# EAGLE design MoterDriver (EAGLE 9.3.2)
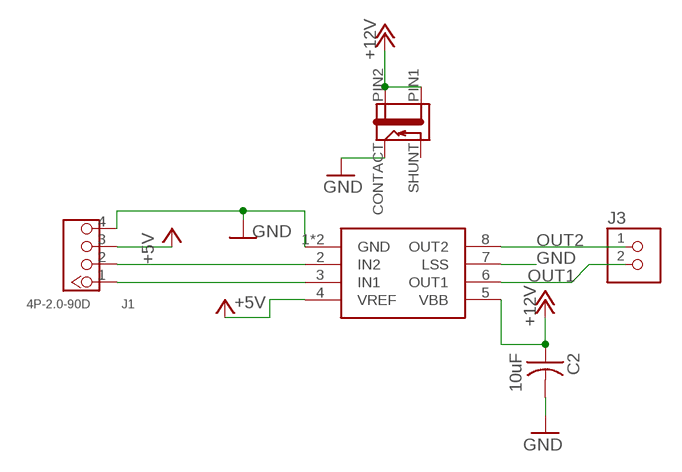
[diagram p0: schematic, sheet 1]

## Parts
C2  10uF  CAP-US1206FAB  [C1206FAB]
J1  4P-2.0-90D  GROVE-CONNECTOR-DIP-90D(4P-2.0)  [HW4-2.0-90D]
J2  JACK-2.1MM  [PJ-002AH-SMT]
J3  TERM-1X02-FABLAB  [ED555DS-2DS]
U$2  A4953-H-BRIDGE-MOTOR-DRIVER-PAD  [SOIC8_PAD]

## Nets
+5V: J1.3 U$2.4(VREF)
+12V: C2.1 J2.PIN1 J2.PIN2 U$2.5(VBB)
GND: C2.2 J1.4 J2.CONTACT U$2.1(GND) U$2.7(LSS) U$2.GND
OUT1: J3.2 U$2.6(OUT1)
OUT2: J3.1 U$2.8(OUT2)
PIN1: J1.1 U$2.3(IN1)
PIN2: J1.2 U$2.2(IN2)

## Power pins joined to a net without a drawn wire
SHUNT: J2.SHUNT

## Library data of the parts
C2 = fab:CAP-US
J1 = OPL_Connector:GROVE-CONNECTOR-DIP-90D(4P-2.0): 320110034
J2 = fab:JACK-2.1MM: SMD DC power jack PJ-002AH-SMT As found in the fablab inventory. Made by Zaerc.
J3 = fab:TERM-1X02: 3.5mm terminal block, 2 positions ED555-2DS as found in the fablab inventory.
U$2 = fab:A4953-H-BRIDGE-MOTOR-DRIVER-PAD

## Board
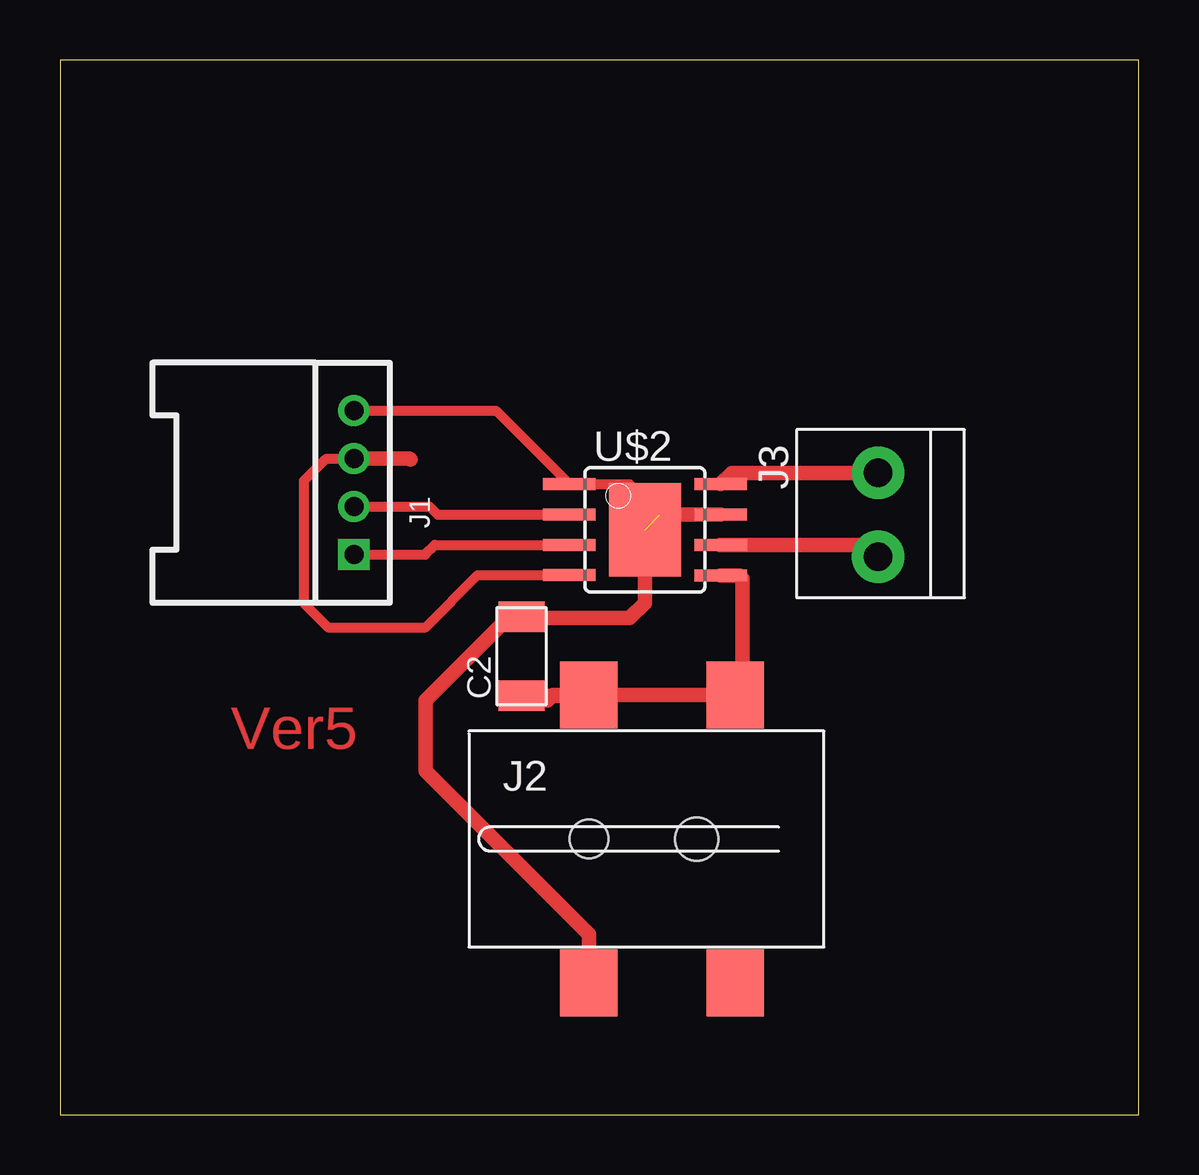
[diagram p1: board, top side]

Size 44.97 x 43.97 mm. Coordinates in mm from the lower left corner, seen from the top.
Outline: 0,0 44.97,0 44.97,43.97 0,43.97 0,0
Copper layers (1*16): Top 0.035mm / dielectric 1.5mm / Bottom 0.035mm
Design rules "default": minimum track width 6mil, minimum drill 0.35mm, track to track 6mil, track to pad 6mil, pad to pad 6mil, via to via 6mil, smd to smd 6mil, copper to edge 40mil, drill to drill 6mil, minimum pad ring 10mil, minimum via ring 8mil, stop-mask expansion 4mil, vias tented up to drill 0mil, thermal gap 10mil

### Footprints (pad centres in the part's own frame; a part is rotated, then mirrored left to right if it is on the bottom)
C1206FAB = smd 1.27 x 1.905: 1 -1.651,0; 2 1.651,0
HW4-2.0-90D = drill 0.8 pad 1.27 square: 1 -3,0 | drill 0.8 pad 1.27: 2 -1,0; 3 1,0; 4 3,0
PJ-002AH-SMT = smd 2.4 x 2.8: CONTACT -2.4,-6; PIN1 3.7,6; PIN2 -2.4,6; SHUNT 3.7,-6 | hole 1.6: -2.4,0 | hole 1.8: 2.1,0
ED555DS-2DS = drill 1.2 pad 2.184: 1 1.8,0; 2 -1.7,0
SOIC8_PAD = smd 0.5 x 2.2: 1 -1.905,-3.154; 2 -0.645,-3.154; 3 0.625,-3.154; 4 1.895,-3.154; 5 1.905,3.154; 6 0.635,3.154; 7 -0.635,3.154; 8 -1.905,3.154 | smd 3.886 x 2.997: GND 0,0

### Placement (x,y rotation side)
C2  19.24,19.11 90 top
J1  12.26,26.35 90 top
J2  24.45,11.49 0 top
J3  34.1,24.96 90 top
U$2  24.38,24.38 270 top

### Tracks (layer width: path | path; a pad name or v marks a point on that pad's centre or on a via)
+5V
  Top 0.406: U$2.4 17.41,22.49 15.24,20.32 11.18,20.32 10.16,21.34 10.16,26.42 11.1,27.35 J1.3
  Top 0.61: J1.3 14.56,27.35 14.61,27.3
+12V
  Top 0.61: U$2.5 28.32,22.48 28.45,22.35 28.45,18.29 | 28.45,17.79 28.45,18.29 | 28.45,18.29 28.15,17.99 J2.PIN1 J2.PIN2 21.34,17.49 | 21.34,17.49 20.54,17.49 20.32,17.27 | C2.1 21.3,17.46 21.34,17.49
GND  (1 unrouted)
  Top 0.406: J1.4 18.17,29.35 U$2.1 23.75,26.29 25.02,25.02
  Top 0.61: J2.CONTACT 22.05,7.53 15.24,14.33 15.24,17.27 18.54,20.57 18.67,20.57 18.86,20.77 C2.2 19.3,20.7 23.75,20.7 24.38,21.34 U$2.GND | 25.02,25.02 U$2.7
OUT1
  Top 0.61: U$2.6 33.61,23.75 J3.2
OUT2
  Top 0.61: U$2.8 28,26.76 J3.1
PIN1
  Top 0.406: J1.1 15.22,23.35 15.63,23.76 U$2.3
PIN2
  Top 0.406: J1.2 15.41,25.35 15.75,25.02 15.76,25.03 U$2.2

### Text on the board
Top: Ver5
